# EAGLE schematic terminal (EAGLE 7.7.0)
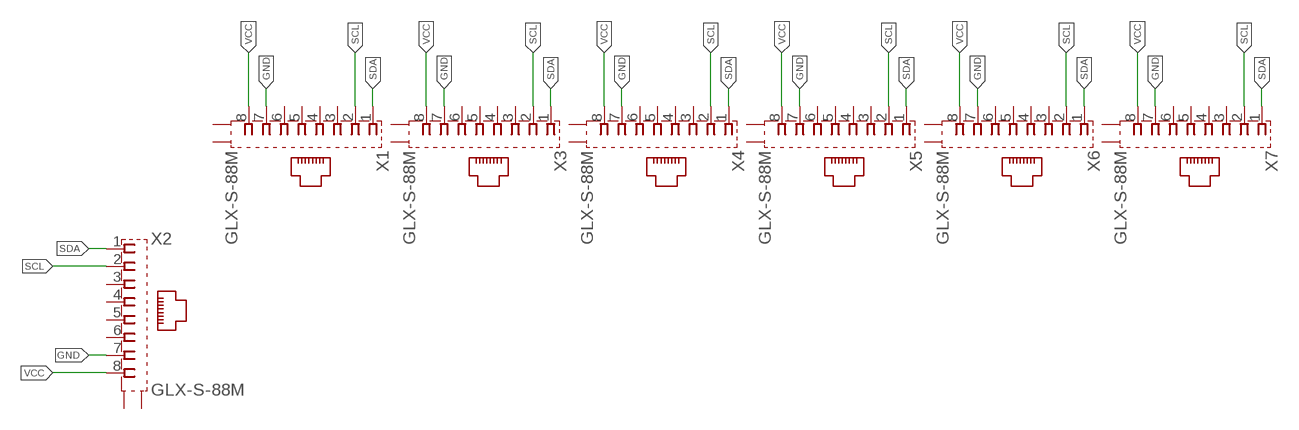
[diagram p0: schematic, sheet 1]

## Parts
X1  GLX-S-88M  [GLX-S-88M]
X2  GLX-S-88M  [GLX-S-88M]
X3  GLX-S-88M  [GLX-S-88M]
X4  GLX-S-88M  [GLX-S-88M]
X5  GLX-S-88M  [GLX-S-88M]
X6  GLX-S-88M  [GLX-S-88M]
X7  GLX-S-88M  [GLX-S-88M]

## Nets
GND: X1.7 X2.7 X3.7 X4.7 X5.7 X6.7 X7.7
SCL: X1.2 X2.2 X3.2 X4.2 X5.2 X6.2 X7.2
SDA: X1.1 X2.1 X3.1 X4.1 X5.1 X6.1 X7.1
VCC: X1.8 X2.8 X3.8 X4.8 X5.8 X6.8 X7.8
Unconnected: X1.3 X1.4 X1.5 X1.6 X1.S1 X1.S2 X2.3 X2.4 X2.5 X2.6 X2.S1 X2.S2 X3.3 X3.4 X3.5 X3.6 X3.S1 X3.S2 X4.3 X4.4 X4.5 X4.6 X4.S1 X4.S2 X5.3 X5.4 X5.5 X5.6 X5.S1 X5.S2 X6.3 X6.4 X6.5 X6.6 X6.S1 X6.S2 X7.3 X7.4 X7.5 X7.6 X7.S1 X7.S2

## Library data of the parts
X1-X7 = con-kycon:GLX-S-88M: Mod. Jack, Right Angle, 8 posiotion, 8 contatcs RJ45 Source: GLX-S-88M.pdf; OC_FARNELL: unknown; OC_NEWARK: unknown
